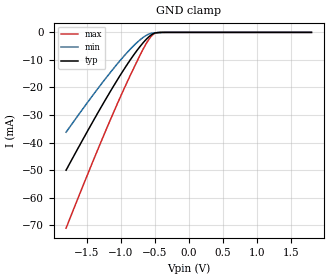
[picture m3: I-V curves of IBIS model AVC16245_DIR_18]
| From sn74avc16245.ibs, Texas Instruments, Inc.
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[Model]   AVC16245_DIR_18
Model_type  Input
Vinl = 0.5775
Vinh = 1.2675
| variable   typ   min   max
C_comp   1.92pF   1.49pF   2.19pF
[Temperature Range]   40   100   -40
| Ambient temperature   25   85   -40
[Voltage range]   1.8   1.65   1.95
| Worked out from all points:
|   GND clamp passes 1 mA (typ) near -0.56 V on its own axis
[GND Clamp]
| AVC16245_DIR_18
|   Voltage   I(typ)   I(min)   I(max)
-1.8V     -50mA      -36.21mA   -71.03mA
-1.345V   -29.67mA   -20.75mA   -43.13mA
-985mV    -14.75mA   -9.574mA   -22.4mA
-805mV    -8.087mA   -4.753mA   -12.84mA
-665mV    -3.636mA   -1.756mA   -5.869mA
-585mV    -1.602mA   -602.7uA   -2.54mA
-520mV    -453.3uA   -219.6uA   -701.3uA
-480mV    -166.9uA   -118.3uA   -185.6uA
-390mV    -15.74uA   -24.31uA   -8.777uA
1.8V      678pA      10.87nA    27.01pA
